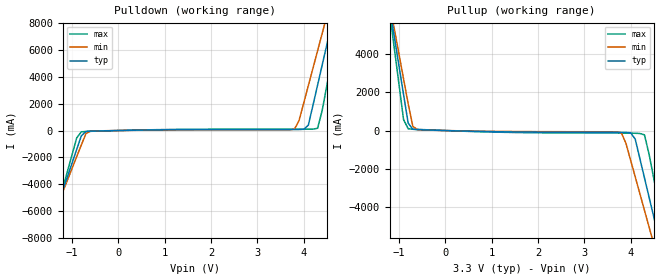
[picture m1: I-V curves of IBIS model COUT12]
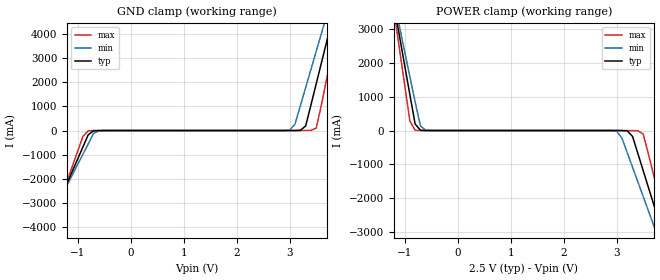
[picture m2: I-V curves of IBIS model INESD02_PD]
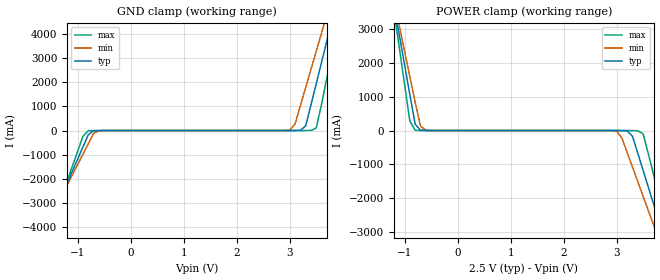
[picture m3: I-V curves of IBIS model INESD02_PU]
|   This file is an IBIS representation of the   |
|   Integrated Device Technology,Inc.   |
|   ICS840002   |
|   LVCMOS/LVTTL Frequency Synthesizer   |
[IBIS Ver]   4.0
[File name]   840002_3v3.ibs
[File Rev]   1.0
[Date]   Dec 17 2007 | Last Modified
|   Dec 17 2007 | Generated
[Source] Originated at Integrated Device Technology,Inc
[Disclaimer]
IDT hereby grants the user of this IBIS model a non-exclusive,
nontransferable license to use this IBIS model under the following terms.
Before using this IBIS model, the user should read this license.
If the user does not accept these terms,  the IBIS model should be
returned to IDT within 30 days.
   The user is granted this license only to use the IBIS model and
is not granted rights to sell, load, rent, lease or license the IBIS
model in whole or in part, or in modified form to anyone other than
user. User may modify the IBIS model to suit its specific
applications but rights to derivative works and such modifications
shall belong to IDT.
   This IBIS model is provided on an "AS IS" basis and IDT makes
absolutely no warranty with respect to the information contained
herein. ICS DISCLAIMS AND CUSTOMER WAIVES ALL WARRANTIES, EXPRESS
OR IMPLIED, INCLUDING WARRANTIES OF MERCHANTABILITY OR FITNESS FOR
A PARTICULAR PURPOSE. The entire risk as to quality and performance
is with the Customer. ACCORDINGLY, IN NO EVENT SHALL THE COMPANY BE
LIABLE FOR ANY DAMAGES, WHETHER IN CONTRACT OR TORT,INCLUDING ANY
LOST PROFITS OR OTHER INCIDENTAL, CONSEQUENTIAL, EXEMPLARY, OR
PUNITIVE DAMAGES ARISING OUT OF THE USE OR APPLICATION OF THE IBIS
model provided in this package. Further, IDT reserves the right to
make changes without notice to any product herein to improve
reliability, function, or design. IDT does not convey any license
under patent rights or any other intellectual property rights,
including those of third parties.
   IDT is not obligated to provide maintenance or support
for the licensed IBIS model.
[Copyright]   Copyright 2007 by Integrated Device Technology,Inc
[Component]   ICS840002AG
[Manufacturer] Integrated Device Technology,Inc
[Package]
|   TSSOP16   typ   min   max
R_pkg   58.65m   52.5m   64.8m
L_pkg   1.902nH   1.443nH   2.361nH
C_pkg   0.315pF   0.254pF   0.375pF
[Pin] signal_name   model_name   R_pin   L_pin   C_pin
1   F_SEL0   INESD02_PU   64.8m   2.361n   0.375p
2   XTAL_SEL   INESD02_PD   60.7m   2.054n   0.335p
3   TEST_CLK   INESD02_PD   56.6m   1.749n   0.294p
4   OE   INESD02_PU   52.5m   1.443n   0.254p
5   MR   INESD02_PD   52.5m   1.443n   0.254p
6   nPLL_SEL   INESD02_PD   56.6m   1.749n   0.294p
7   VDDA   POWER   60.7m   2.054n   0.335p
8   VDD   POWER   64.8m   2.361n   0.375p
9   XTAL_OUT   NC   64.8m   2.361n   0.375p
10   XTAL_IN   NC   60.7m   2.054n   0.335p
11   VDDO   POWER   56.6m   1.749n   0.294p
12   Q1   COUT12   52.5m   1.443n   0.254p
13   Q0   COUT12   52.5m   1.443n   0.254p
14   GND   GND   56.6m   1.749n   0.294p
15   GND   GND   60.7m   2.054n   0.335p
16   FSEL1   INESD02_PU   64.8m   2.361n   0.375p
| Models and submodels in the file (3): COUT12 (Output), INESD02_PD (Input), INESD02_PU (Input)
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[Model]   COUT12
Model_type   Output
Polarity   Non-Inverting
Vmeas = 1.65
Rref = 50
Cref = 0
Vref = 1.65
|   typ   min   max
C_comp   2pF   1.5pF   2.5pF
|   typ   min   max
[Voltage range]  3.3V   3.15V   3.45V
|   typ   min   max
[Temperature Range]   27.0   -40   85
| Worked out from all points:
|   slope of the pulldown table from 0 to 0.495 V, typ, clamps not added: 15.4 ohm
|   slope of the pullup table from 0 to 0.495 V, typ, clamps not added: 15.2 ohm
[pulldown]
|Voltage   I (typ)   I (min)   I (max)
-3.3V     -25.76A    -22.97A    -30.46A
-1.5V     -7.499A    -7.2A      -8.039A
-900mV    -1.412A    -1.95A     -555.6mA
-800mV    -399.2mA   -1.076A    -95.23mA
-600mV    -44.85mA   -44.17mA   -58.2mA
3.8V      74.94mA    98.59mA    96.98mA
4.1V      400.7mA    3.343A     99.24mA
4.3V      3.388A     5.943A     169.6mA
4.4V      4.894A     7.244A     1.513A
4.6V      7.909A     9.846A     5.22A
4.8V      10.93A     12.45A     8.931A
6.6V      38.21A     35.99A     42.48A
[pullup]
|Voltage   I (typ)   I (min)   I (max)
-3.3V     38.17A     34.02A     45.19A
-1.2V     6.403A     6.598A     6.145A
-1.1V     4.892A     5.294A     4.286A
-900mV    1.87A      2.687A     569.6mA
-800mV    383.2mA    1.384A     89.62mA
-600mV    45.84mA    44mA       59.23mA
3.8V      -96.26mA   -112.7mA   -131.6mA
4.1V      -444.3mA   -2.407A    -142.4mA
4.3V      -2.464A    -4.151A    -227.1mA
4.6V      -5.499A    -6.77A     -3.731A
4.8V      -7.524A    -8.517A    -6.22A
6.6V      -25.76A    -24.26A    -28.62A
[Ramp]
|   typ   min   max
dV/dt_r   1.98/0.6n   1.98/0.80n   1.98/0.4n
dV/dt_f   1.98/0.6n   1.98/0.80n   1.98/0.4n
[Model]   INESD02_PD
Model_type   Input
Polarity   Non-Inverting
Vinl = 1.4V
Vinh = 1.85V
|   typ   min   max
C_comp   2pF   1.5pF   2.5pF
|   typ   min   max
[Voltage range]  2.5V   2.375V   2.625V
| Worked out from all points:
|   GND clamp passes 1 mA (typ) near -0.55 V on its own axis
|   POWER clamp passes 1 mA (typ) near -0.60 V on its own axis
[GND_clamp]
|Voltage I(typ)   I(min)   I(max)
-2.5V     -8.775A    -7.892A    -10.18A
-1.6V     -4.218A    -4.001A    -4.586A
-900mV    -678.5mA   -979.3mA   -237.6mA
-800mV    -173.9mA   -548.7mA   -10.83mA
-600mV    -1.629mA   -8.74mA    -911.1uA
3V        133.3uA    17.16mA    56.6uA
3.1V      660.9uA    273.5mA    60.87uA
3.3V      191.6mA    1.785A     327.9uA
3.5V      1.949A     3.298A     103.6mA
3.7V      3.723A     4.812A     2.189A
3.9V      5.498A     6.327A     4.369A
5V        15.27A     14.67A     16.38A
[POWER_clamp]
|Voltage   I(typ)   I(min)   I(max)
-2.5V     15.27A     13.72A     17.74A
-1.2V     3.723A     3.866A     3.551A
-1.1V     2.836A     3.109A     2.461A
-900mV    1.063A     1.596A     283.3mA
-800mV    191.6mA    840.1mA    6.189mA
-600mV    660.9uA    8.845mA    114.2uA
3V        -338.1uA   -16.36mA   -12.68uA
3.4V      -678.5mA   -1.518A    -7.183mA
3.5V      -1.183A    -1.95A     -99.52mA
3.7V      -2.195A    -2.813A    -1.324A
4V        -3.712A    -4.109A    -3.188A
5V        -8.775A    -8.432A    -9.404A
[Model]   INESD02_PU
Model_type   Input
Polarity   Non-Inverting
Vinl = 1.4V
Vinh = 1.85V
|   typ   min   max
C_comp   2pF   1.5pF   2.5pF
|   typ   min   max
[Voltage range]  2.5V   2.375V   2.625V
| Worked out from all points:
|   GND clamp passes 1 mA (typ) near -0.55 V on its own axis
|   POWER clamp passes 1 mA (typ) near -0.61 V on its own axis
[GND_clamp]
|Voltage   I(typ)   I(min)   I(max)
-2.5V     -8.775A    -7.892A    -10.18A
-1.6V     -4.218A    -4.001A    -4.586A
-900mV    -678.5mA   -979.4mA   -237.6mA
-800mV    -173.9mA   -548.7mA   -10.88mA
-600mV    -1.682mA   -8.796mA   -960.5uA
3V        79.39uA    17.1mA     7.198uA
3.1V      607uA      273.4mA    11.46uA
3.3V      191.5mA    1.785A     278.5uA
3.5V      1.949A     3.298A     103.5mA
3.7V      3.723A     4.812A     2.189A
3.9V      5.498A     6.327A     4.369A
5V        15.27A     14.67A     16.38A
[POWER_clamp]
|Voltage   I(typ)   I(min)   I(max)
-2.5V     15.27A     13.72A     17.74A
-1.2V     3.723A     3.866A     3.551A
-1.1V     2.836A     3.109A     2.461A
-900mV    1.063A     1.596A     283.3mA
-800mV    191.5mA    840mA      6.139mA
-600mV    607uA      8.789mA    64.82uA
3V        -392uA     -16.42mA   -62.09uA
3.4V      -678.5mA   -1.518A    -7.233mA
3.5V      -1.184A    -1.95A     -99.57mA
3.7V      -2.195A    -2.813A    -1.324A
4V        -3.712A    -4.109A    -3.188A
5V        -8.775A    -8.433A    -9.404A
